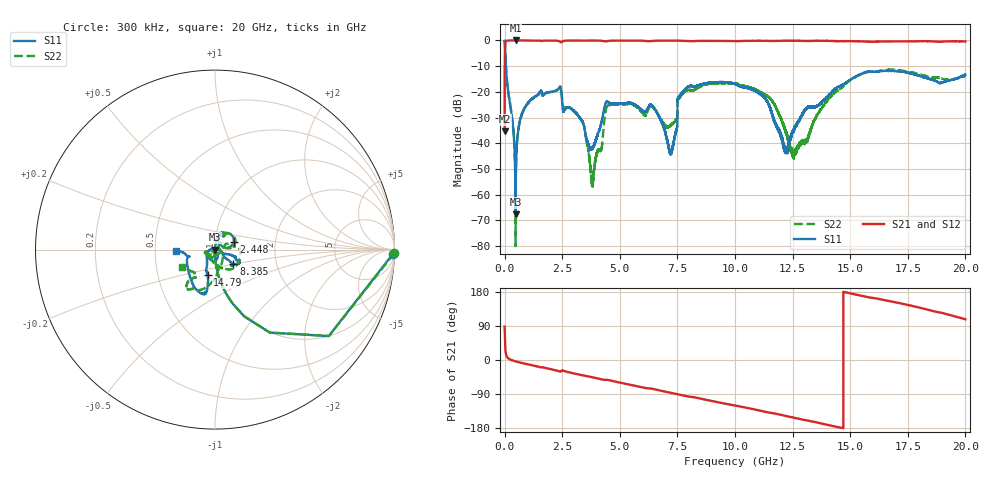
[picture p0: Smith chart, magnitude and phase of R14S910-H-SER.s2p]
!{R14S910}
!Johanson Technology Inc.
!www.johansontechnology.com
!Test Board Conditions:
!Substrate Type  RO4350B
!Substrate Thickness  20 mil
!Substrate Dk  3.66
!TL Type: GCPW
!TL Trace Width  36 mil
!TL Gap  12 mil
!Electrode orientation  Horizontal
!DUT TOPOLOGY	SERIES
!Mounting Pad LxW  26x36 mil
! Created Wed Nov 25 17:33:21 2020
! 2 Port Network Data from SP1.SP block
! freq  magS11  angS11  magS21  angS21  magS12  angS12  magS22  angS22
# khz S ma R 50
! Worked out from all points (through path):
!   20001 points, 300 kHz to 20 GHz, reference 50 ohm
!   highest |S21| = 0.00 dB at 473.3 MHz (marker M1); lowest = -35.3 dB at 300 kHz (marker M2)
!   group delay of S21, straight-line fit = 34.7 ps
!   lowest |S11| = -67.7 dB at 476.3 MHz (marker M3), VSWR 1.00, Z = 50 + j0.0285 ohm
!   |S11| at or under -10 dB: 51.99 MHz to end of sweep
!   |S22| runs from -80.1 to 0.0 dB; largest |S21 - S12| = 0.017
!   S11 on the Smith chart (normalised r, x): 300 kHz: 26, -82; 2.448 GHz: 1.23, +0.11; 8.385 GHz: 1.21, -0.20; 14.79 GHz: 0.89, -0.26; 20 GHz: 0.64, -0.01
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300  0.993 -1.3  0.01711 87.9  0.01711 88.6  0.9982 -1.1
108300  0.1527 -82.0  0.9876 7.9  0.9879 7.9  0.1534 -82.0
473300  0.0005859 -144.5  1 -3.5  0.9989 -3.5  0.0003451 -54.4
476300  0.0004116 136.1  0.9992 -3.7  1 -3.6  9.899e-05 72.6
691300  0.03022 84.0  0.9986 -7.0  0.9989 -7.0  0.03023 82.4
1009300  0.06003 79.3  0.9977 -11.5  0.9976 -11.4  0.05993 77.9
2448300  0.1128 22.3  0.9213 -29.6  0.9212 -29.6  0.121 19.4
3334300  0.02818 45.0  0.9951 -39.7  0.9959 -39.7  0.02829 39.6
3808300  0.007878 -37.3  0.9962 -45.6  0.9964 -45.6  0.001796 134.4
4499300  0.06261 -112.3  0.9782 -52.8  0.9777 -52.8  0.05479 -136.6
6667300  0.0355 -168.6  0.9903 -79.4  0.9898 -79.4  0.03565 -146.5
7224300  0.006535 98.2  0.9902 -86.7  0.9909 -86.7  0.02272 -81.7
7600300  0.08396 -37.9  0.9879 -91.6  0.9883 -91.6  0.07873 25.2
8385300  0.1312 -38.6  0.9789 -100.4  0.9786 -100.4  0.12 9.7
1.00003e7  0.1426 -26.1  0.9718 -120.2  0.9717 -120.3  0.1456 -46.5
1.13173e7  0.07516 -20.7  0.983 -136.7  0.9832 -136.7  0.08665 -82.2
1.22083e7  0.00835 86.1  0.9878 -147.6  0.9908 -147.7  0.01643 -143.8
1.25733e7  0.0192 166.2  0.9864 -152.5  0.9871 -152.5  0.006587 116.2
1.33343e7  0.04991 -164.7  0.9797 -161.8  0.9813 -161.8  0.02117 15.4
1.47943e7  0.1481 -106.1  0.9721 178.8  0.9716 178.6  0.1423 -86.5
1.66673e7  0.2541 -105.2  0.9598 155.8  0.9533 155.6  0.2688 -124.1
2e7  0.2164 -177.7  0.9572 107.6  0.9547 107.7  0.2074 -151.8
